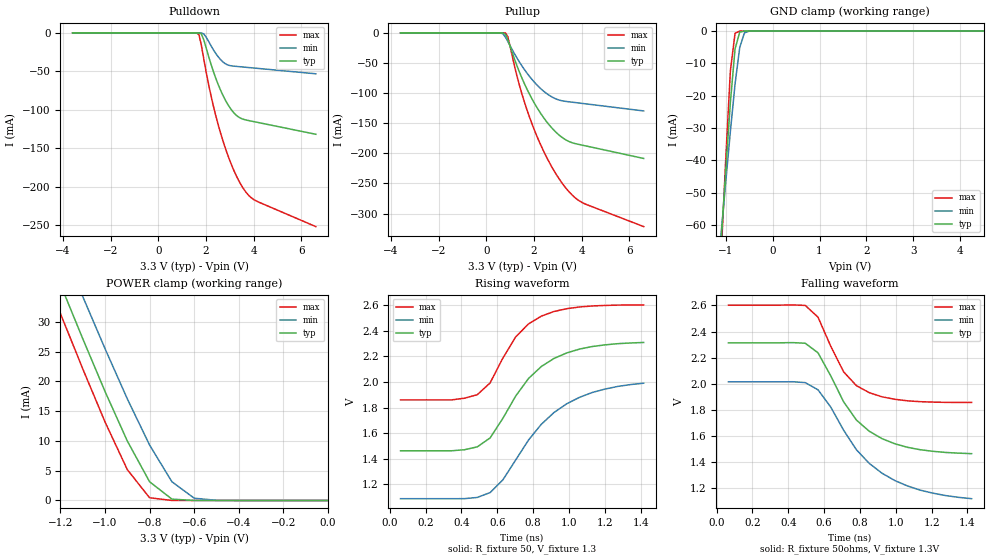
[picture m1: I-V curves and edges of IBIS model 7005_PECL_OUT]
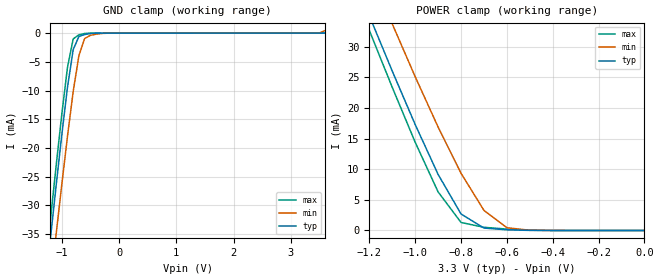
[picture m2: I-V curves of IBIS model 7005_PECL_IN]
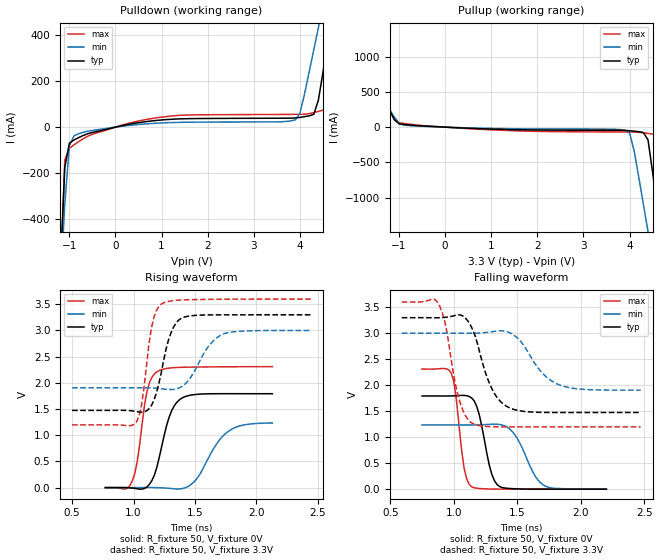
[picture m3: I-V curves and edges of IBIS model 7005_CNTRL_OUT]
|   This file is an IBIS representation of the   |
|   Texas Instruments   |
|   CDC7005   |
|   64 CABGA Package   |
[IBIS Ver]   3.2
[File name]   cdc7005x_02.ibs
[File Rev]   0.2
[Date]   18th of Feb 2004
[Source]   file originated at Texas Instruments
[Notes]   The following information corresponds to the
|   CDC7101 input/output buffers and input ESD structures.
|Revision log: 0.1, 10/02/2002 file released by TEXAS INSTRUMENTS.
|   1- initial version
|   0.2, 02/18/2004 replaced GND Clamp (referenced to VDD), with
|   same plot referenced to GND (0V).
|   Warnings for VT/IV voltage difference relate to truncated
|   VT plots to allow faster simulation frequency if
|   VT time delay is enabled, which is strongly recommended for
|   correct results of the differential PECL buffers. If this is not
|   required, some simulators require to completely disable use of
|   the VT table for better results. If you note problems with
|   differential cross point, it might point to this situation !
[Disclaimer]
(C) Copyright Texas Instruments Incorporated 2001
   All rights reserved
  Texas Instruments Incorporated hereby grants the user of this IBIS
model a non-exclusive, nontransferable license to use this IBIS model
under the following terms.  Before using this IBIS model, the user
should read this license.  If the user does not accept these terms,
the IBIS model should be returned to Texas Instruments within 30 days.
  The user is granted this license only to use the IBIS model and
is not granted rights to sell, load, rent, lease or license the IBIS
model in whole or in part, or in modified form to anyone other than
user.  User may modify the IBIS model to suit its specific applications
but rights to derivative works and such modifications shall belong to
Texas Instruments.
  This IBIS model is provided on an "AS IS" basis and Texas Instruments
makes absolutely no warranty with respect to the information contained
herein.  TEXAS INSTRUMENTS DISCLAIMS AND CUSTOMER WAIVES ALL WARRANTIES,
EXPRESS OR IMPLIED, INCLUDING WARRANTIES OF MERCHANTABILITY OR FITNESS
FOR A PARTICULAR PURPOSE. The entire risk as to quality and performance
is with the Customer. ACCORDINGLY, IN NO EVENT SHALL THE COMPANY BE LIABLE
FOR ANY DAMAGES, WHETHER IN CONTRACT OR TORT,INCLUDING ANY LOST PROFITS
OR OTHER INCIDENTAL, CONSEQUENTIAL, EXEMPLARY, OR PUNITIVE DAMAGES ARISING
OUT OF THE USE OR APPLICATION OF THE IBIS model provided in this package.
Further, Texas Instruments reserves the right to discontinue or make changes
without notice to any product herein to improve reliability, function, or
design. Texas Instruments does not convey any license under patent rights
or any other intellectual property rights, including those of third parties.
Contact Texas Instruments at ATTN: HPA Department,
12500 TI blvd, M/S 8730, Dallas, TX 75243
IBIS Open Forum disclaims all warranties. See DISCLAIM.TXT
in vhdl.org:/pub/IBIS/models for the full disclaimer.
[Copyright]   Copyright 2002, Texas Instruments, All Rights Reserved
[Component]   CDC7005ZVA
[Manufacturer]  Texas Instruments Incorporated
[Package]
| Package paracitics for signal pins only
|   TYP   MIN   MAX
R_pkg   0.197ohms   0.117ohms   0.222ohms
L_pkg   1.790nH   1.335nH   2.000nH
C_pkg   0.600pF   0.506pF   0.675pF
[Pin]   signal_name   model_name   R_Pin   L_Pin   C_Pin
A1   CTRL_LE   7005_SPI_IN   0.200ohms   1.746nH   0.606pF
A2   CTRL_CLK   7005_SPI_IN   0.222ohms   2.000nH   0.597pF
A3   CTRL_DATA   7005_SPI_IN   0.204ohms   1.836nH   0.636pF
A4   CP_OUT   7005_CP_OUT   0.117ohms   1.335nH   0.606pF
A5   OPA_IN   7005_OPA_IN   0.198ohms   1.820nH   0.566pF
A6   OPA_IP   7005_OPA_IN   0.204ohms   1.875nH   0.560pF
A7   OPA_OUT   7005_OPA_OUT   0.134ohms   1.467nH   0.570pF
A8   STATUS_LOCK   7005_CNTRL_OUT   0.199ohms   1.704nH   0.609pF
B1   REF_IN   7005_REF_IN   0.221ohms   1.944nH   0.506pF
|C1   I_REF   7005_IREF   0.203ohms   1.866nH   0.614pF
C8   STATUS_REF   7005_CNTRL_OUT   0.205ohms   1.826nH   0.556pF
D1   VCXO_IN   7005_PECL_IN   0.197ohms   1.803nH   0.675pF
D8   STATUS_VCOX   7005_CNTRL_OUT   0.195ohms   1.763nH   0.557pF
E1   VCXO_IN_B   7005_PECL_IN   0.200ohms   1.826nH   0.658pF
F1   Y0   7005_PECL_OUT   0.206ohms   1.854nH   0.600pF
F8   Y4B   7005_PECL_OUT   0.202ohms   1.849nH   0.601pF
G1   Y0B   7005_PECL_OUT   0.211ohms   1.886nH   0.607pF
G8   Y4   7005_PECL_OUT   0.208ohms   1.767nH   0.522pF
H1   NPD   7005_LOGIC_IN   0.199ohms   1.736nH   0.604pF
H2   Y1   7005_PECL_OUT   0.205ohms   1.874nH   0.638pF
H3   Y1B   7005_PECL_OUT   0.189ohms   1.736nH   0.606pF
H4   Y2   7005_PECL_OUT   0.200ohms   1.835nH   0.623pF
H5   Y2B   7005_PECL_OUT   0.201ohms   1.843nH   0.607pF
H6   Y3   7005_PECL_OUT   0.204ohms   1.882nH   0.619pF
H7   Y3B   7005_PECL_OUT   0.208ohms   1.898nH   0.647pF
H8   NRESET   7005_LOGIC_IN   0.203ohms   1.571nH   0.601pF
| equivilant summary for balls: C3,C4,C5,C6,C7 and C7
C3   AVCC_all   Power   0.034ohms   0.319nH   2.076pF
| equivilant summary for balls: B2,B3,B4,B5,B6,B7,B8,C2,D2,D3,D4,D5,D6
|   E2,F2,F3,F4,F5,F6
B2   GND_all   GND   0.008ohms   0.069nH   7.236pF
| equivilant summary for balls: D7,E3,E4,E5,E6,E7,E8,F7,G2,G3,G4,G5,G6,G7
D7   VCC_all   Power   0.011ohms   0.099nH   4.810pF
[Diff_Pin]  inv_pin  vdiff   tdelay_typ  tdelay_min  tdelay_max
F1   G1   0V   0ns   0ns   0ns   | Y0+ / Y0-
H2   H3   0V   0ns   0ns   0ns   | Y1+ / Y1-
H4   H5   0V   0ns   0ns   0ns   | Y2+ / Y2-
H6   H7   0V   0ns   0ns   0ns   | Y3+ / Y3-
G8   F8   0V   0ns   0ns   0ns   | Y4+ / Y4-
D1   E1   0.5V   0ns   0ns   0ns   | VCXO_IN+ / VCXO_IN-
A6   A5   0.1V   0ns   0ns   0ns   | OPA_IP / OPA_IN
[Model Selector]   7005_CP_OUT
7005_CP_DOWN   negative_pulse_2mA
7005_CP_UP   positive_pulse_2mA
| Models and submodels in the file (10): 7005_PECL_OUT (3-state_ECL), 7005_PECL_IN (Input), 7005_CNTRL_OUT (Output), 7005_REF_IN (Input), 7005_SPI_IN (Input), 7005_LOGIC_IN (Input), 7005_OPA_OUT (Output), 7005_OPA_IN (Input), 7005_CP_UP (3-state), 7005_CP_DOWN (3-state)
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|   Differential Output Driver MODEL
[Model]   7005_PECL_OUT
Model_type   3-state_ECL
| Signals   Y0, Y0B, Y1, Y1B, Y2, Y2B, Y3, Y3B, Y4, Y4B
Vmeas = 1.89V   |Vref for timing measurments
Cref = 0pF   |c_load for timing spec
Rref = 50   |R_load for timing spec
Vref = 1.3V   |Timing spec test load voltage
| variable   typ   min   max
C_comp   1.6pF   1.2pF   2.2pF
[Temperature Range]   27   125   -20
[Voltage range]   3.3V   3.0V   3.6V
[Pulldown reference]   3.3V   3.0V   3.6V
[GND Clamp reference]   0V   0V   0V
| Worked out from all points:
|   GND clamp passes 1 mA (typ) near -0.71 V on its own axis
|   POWER clamp passes 1 mA (typ) near -0.73 V on its own axis
|   rising waveform, R_fixture 50, V_fixture 1.3: 20-80 % time 275ps typ, 321ps min, 209ps max; typ from 1.46 V to 2.31 V
|   falling waveform, R_fixture 50ohms, V_fixture 1.3V: 20-80 % time 251ps typ, 314ps min, 183ps max; typ from 2.31 V to 1.47 V
[Pullup]
|   27C:3.3V:nominal   125C:3.0V:weak   -20C:3.6V:strong
|  Voltage   I(typ)   I(min)   I(max)
-3.6V     437pA      8.06nA     324.7pA
500mV     -84.04nA   -11.65uA   -371.3pA
700mV     -101.2uA   -1.872mA   -2.864uA
800mV     -2.246mA   -7.123mA   -226.3uA
900mV     -11.06mA   -14.21mA   -6.425mA
1.4V      -66.31mA   -49.24mA   -88.69mA
1.9V      -108.6mA   -76.68mA   -149.5mA
2.5V      -146mA     -99.87mA   -204.2mA
3.2V      -174.2mA   -112.9mA   -250.6mA
3.6V      -182.4mA   -115.1mA   -269.2mA
4V        -186.2mA   -117mA     -281.2mA
6.6V      -208.5mA   -129.6mA   -321.5mA
[Pulldown]
|   27C:3.3V:nominal   125C:3.0V:weak   -20C:3.6V:strong
|   Voltage   I(typ)   I(min)   I(max)
-3.6V     280.9pA    304.5pA    264.7pA
1.6V      -1.679uA   -521.3nA   -43.83uA
1.7V      -58.05uA   -8.476uA   -2.396mA
1.8V      -1.47mA    -132uA     -16mA
1.9V      -8.843mA   -1.407mA   -33.6mA
2.2V      -40.32mA   -16.53mA   -81.03mA
2.5V      -66.73mA   -30.89mA   -118.8mA
3V        -97.48mA   -42.66mA   -166.6mA
3.5V      -111.8mA   -44.34mA   -199.5mA
3.8V      -114.3mA   -45.21mA   -211.9mA
4.1V      -116.2mA   -46.08mA   -218.7mA
6.6V      -132mA     -53.32mA   -252.1mA
[GND Clamp]
|   27C:3.3V:nominal   125C:3.0V:weak   -20C:3.6V:strong
|   Voltage   I(typ)   I(min)   I(max)
-3.6V     -846.1mA   -726mA     -1.01A
-1.1V     -65.74mA   -63.12mA   -70.56mA
-1V       -43.58mA   -46.98mA   -40.08mA
-900mV    -22.15mA   -31.16mA   -12.38mA
-800mV    -5.529mA   -16.41mA   -692.9uA
-700mV    -333.5uA   -5.056mA   -8.688uA
-600mV    -9.161uA   -575uA     -94.39nA
-500mV    -237.2nA   -35.55uA   -1.21nA
6.6V      452.4pA    471.7pA    424.6pA
[POWER Clamp]
|   27C:3.3V:nominal   125C:3.0V:weak   -20C:3.6V:strong
|  Voltage   I(typ)   I(min)   I(max)
-3.6V     263.5mA    264.3mA    263.5mA
-1.3V     45.57mA    52.26mA    40.83mA
-1.2V     36.3mA     43.2mA     31.38mA
-1.1V     27.17mA    34.25mA    22.11mA
-1V       18.31mA    25.49mA    13.19mA
-900mV    9.992mA    17.07mA    5.178mA
-800mV    3.144mA    9.308mA    454.2uA
-700mV    228.8uA    3.147mA    5.697uA
-600mV    6.116uA    387.4uA    58.55nA
-500mV    150.9nA    23.42uA    752.7pA
0V        84.38pA    102.7pA    89.81pA
[ramp]
| variable   typ   min   max
dV/dt_r   0.5117/2.7842E-10   0.5571/3.3895E-10   0.4456/2.0819E-10
dV/dt_f   0.5117/2.5529E-10   0.5571/3.4568E-10   0.4456/1.8152E-10
[Rising Waveform]
R_fixture = 50
V_fixture =  1.3
V_fixture_min = 1.0
V_fixture_max = 1.6  | Plot was truncated to
|   allow shorter simulation periodes.
|   27C:3.3V:nominal   125C:3.0V:weak  -20C:3.6V:strong
|   Time   V(typ)   V(min)   V(max)
59.71ps   1.462V     1.087V     1.86V
416.9ps   1.47V      1.087V     1.873V
488.3ps   1.492V     1.096V     1.901V
559.7ps   1.562V     1.134V     1.993V
631.1ps   1.716V     1.234V     2.188V
702.6ps   1.89V      1.39V      2.353V
845.4ps   2.121V     1.669V     2.515V
916.9ps   2.185V     1.762V     2.552V
1.06ns    2.258V     1.881V     2.588V
1.417ns   2.31V      1.991V     2.603V
[Falling Waveform]
R_fixture = 50ohms
V_fixture =  1.3V
V_fixture_min = 1.0V
V_fixture_max = 1.6V   |  Plot was truncated to
|   allow shorter simulation periodes.
|   27C:3.3V:nominal   125C:3.0V:weak -20C:3.6V:strong
|   Time   V(typ)   V(min)   V(max)
65.71ps   2.314V     2.015V     2.602V
494.3ps   2.311V     2.01V      2.6V
565.7ps   2.238V     1.955V     2.51V
637.1ps   2.061V     1.822V     2.287V
708.6ps   1.863V     1.645V     2.092V
780ps     1.723V     1.496V     1.987V
922.9ps   1.581V     1.316V     1.901V
1.066ns   1.514V     1.218V     1.87V
1.209ns   1.484V     1.163V     1.86V
1.423ns   1.466V     1.121V     1.858V
|   Differential Input Receiver Model
[Model]   7005_PECL_IN
Model_type   Input
Polarity   Non-Inverting
Enable   Active-High
Vinl = 1.6575V   | PECL levels refer to VDD. 3.3-(1.81+1.475)/2
Vinh = 2.2775V   |   3.3-(1.165+.088)/2
|   typ   min   max
C_comp   0.21pF   NA   NA
[Temperature range]   27   125   -20
[Voltage range]   3.3   3.0   3.6
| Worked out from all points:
|   GND clamp passes 1 mA (typ) near -0.72 V on its own axis
|   POWER clamp passes 1 mA (typ) near -0.73 V on its own axis
| Notes: (1) Vtable = Vcc - Voutput
|   (2) Pullup data includes the effects of the clamping circuitry
[POWER Clamp]
|   27C:3.3V:nominal   125C:3.0V:weak   -20C:3.6V:strong
|  Voltage   I(typ)   I(min)   I(max)
-3.6V     265.8mA    263.4mA    273.1mA
-1.2V     35.02mA    42.56mA    32.64mA
-1.1V     26mA       33.7mA     23.35mA
-1V       17.28mA    25.09mA    14.39mA
-900mV    9.15mA     16.88mA    6.291mA
-800mV    2.691mA    9.338mA    1.306mA
-700mV    397uA      3.282mA    517.8uA
-600mV    106.3uA    454.8uA    227uA
-500mV    15.87uA    36.77uA    48.73uA
0V        85.66pA    160pA      90.57pA
[GND Clamp]
|   27C:3.3V:nominal   125C:3.0V:weak   -20C:3.6V:strong
|  Voltage   I(typ)   I(min)   I(max)
-3.6V     -268.1mA   -268.4mA   -271.2mA
-1.3V     -45.38mA   -53.26mA   -42.38mA
-1.2V     -35.99mA   -44.19mA   -32.76mA
-1.1V     -26.76mA   -35.23mA   -23.31mA
-1V       -17.81mA   -26.44mA   -14.21mA
-900mV    -9.461mA   -17.98mA   -5.998mA
-800mV    -2.874mA   -10.17mA   -1.017mA
-700mV    -575.1uA   -3.894mA   -292.2uA
-600mV    -252.8uA   -947.5uA   -69.37uA
-300mV    -10.26uA   -59.25uA   -7.753uA
3.4V      131.5pA    2.975uA    79.13pA
3.6V      47.15nA    454.8uA    90.57pA
|   Device Control Output Driver Model
[Model]   7005_CNTRL_OUT
Model_type   Output
Polarity   Non-Inverting
Enable   Active-High
Vmeas = 0.9V   |Vref for timing measurements.
Cref = 0pF   |load capacitance for timing spec.
Rref = 50ohms   |50 Ohm to GND (VCC)
Vref = 0V   |Timing specification test load voltage; GND
|   typ   min   max
C_comp   1.84pF   NA   NA
[Temperature range]   27   125   -20
[Voltage range]   3.3   3.0   3.6
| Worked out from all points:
|   slope of the pulldown table from 0 to 0.495 V, typ, clamps not added: 25.5 ohm
|   slope of the pullup table from 0 to 0.495 V, typ, clamps not added: 32.4 ohm
|   rising waveform, R_fixture 50, V_fixture 0V: 20-80 % time 119ps typ, 192ps min, 83.9ps max; typ from 0 V to 1.79 V
|   falling waveform, R_fixture 50, V_fixture 0V: 20-80 % time 90.9ps typ, 146ps min, 64.9ps max; typ from 1.79 V to 0 V
|   rising waveform, R_fixture 50, V_fixture 3.3V: 20-80 % time 112ps typ, 171ps min, 81.9ps max; typ from 1.47 V to 3.3 V
|   falling waveform, R_fixture 50, V_fixture 3.3V: 20-80 % time 150ps typ, 200ps min, 110ps max; typ from 3.3 V to 1.48 V
| Notes: (1) Vtable = Vcc - Voutput
|   (2) Pullup data includes the effects of the ESD
|   clamping circuitry
[Pullup]
|   27C:3.3V:nominal   125C:3.0V:weak   -20C:3.6V:strong
|  Voltage   I(typ)   I(min)   I(max)
-3.6V     3.231A     2.546A     4.154A
-2.5V     1.856A     1.489A     2.366A
-2.2V     1.481A     1.2A       1.879A
-1.9V     1.106A     911.7mA    1.391A
-1V       46.45mA    58.48mA    62.25mA
3.9V      -46.72mA   -42.31mA   -68.83mA
4.1V      -57.23mA   -338.9mA   -70mA
4.4V      -181.6mA   -1.482A    -89.55mA
4.6V      -1.142A    -2.251A    -112mA
4.7V      -1.642A    -2.636A    -160.1mA
4.9V      -2.642A    -3.405A    -1.365A
6.6V      -11.14A    -9.943A    -12.41A
[Pulldown]
|   27C:3.3V:nominal   125C:3.0V:weak   -20C:3.6V:strong
|  Voltage   I(typ)   I(min)   I(max)
-3.6V     -12.64A    -9.941A    -16.3A
-1.2V     -638mA     -710.4mA   -698.9mA
-1.1V     -176.9mA   -336.1mA   -142.9mA
-1V       -69.89mA   -80.95mA   -92.23mA
-900mV    -56.15mA   -37.94mA   -77.1mA
900mV     29.4mA     17.24mA    40.92mA
3.9V      40.02mA    31.45mA    55.55mA
4V        42.48mA    60.4mA     55.69mA
4.4V      117.5mA    432.9mA    68.4mA
4.7V      489.8mA    721.3mA    115.4mA
4.9V      739.8mA    913.6mA    433.4mA
6.6V      2.865A     2.548A     3.196A
[ramp]
| variable   typ   min   max
dV/dt_r   1.0759/1.1902E-10   0.7405/1.9176E-10   1.3856/8.3905E-11
dV/dt_f   1.0759/9.0932E-11   0.7405/1.4575E-10   1.3856/6.4836E-11
[Rising Waveform]
R_fixture = 50
V_fixture = 0V
|   27C:3.3V:nominal   125C:3.0V:weak  -20C:3.6V:strong
|   Time   V(typ)   V(min)   V(max)
770.2ps   -100uV     0V         1mV
990.2ps   -9mV       300uV      127.7mV
1.03ns    -20.3mV    800uV      498mV
1.11ns    14.6mV     2mV        1.841V
1.19ns    391.7mV    -400uV     2.211V
1.29ns    1.346V     -13mV      2.282V
1.39ns    1.704V     -21.2mV    2.297V
1.51ns    1.779V     157.1mV    2.302V
1.77ns    1.793V     1.072V     2.307V
2.13ns    1.793V     1.234V     2.309V
[Falling Waveform]
R_fixture = 50
V_fixture = 0V
|   27C:3.3V:nominal   125C:3.0V:weak  -20C:3.6V:strong
|   Time   V(typ)   V(min)   V(max)
750ps     1.793V     1.236V     2.31V
980ps     1.794V     1.236V     2.235V
1.02ns    1.798V     1.235V     1.724V
1.08ns    1.804V     1.235V     419.2mV
1.14ns    1.756V     1.235V     46.3mV
1.2ns     1.433V     1.238V     13.9mV
1.3ns     277.9mV    1.25V      2.6mV
1.36ns    50.6mV     1.244V     1.1mV
1.7ns     600uV      87.7mV     300uV
2.2ns     200uV      500uV      300uV
[Rising Waveform]
R_fixture = 50
V_fixture =  3.3V
V_fixture_min = 3.0
V_fixture_max = 3.6
|   27C:3.3V:nominal   125C:3.0V:weak  -20C:3.6V:strong
|   Time   V(typ)   V(min)   V(max)
500ps     1.474V     1.905V     1.198V
1.025ns   1.452V     1.906V     1.258V
1.065ns   1.441V     1.906V     1.575V
1.145ns   1.565V     1.903V     3.036V
1.185ns   1.8V       1.897V     3.373V
1.245ns   2.425V     1.882V     3.528V
1.325ns   3.061V     1.875V     3.571V
1.405ns   3.25V      1.949V     3.584V
1.725ns   3.299V     2.927V     3.596V
2.445ns   3.299V     3.001V     3.6V
[Falling Waveform]
R_fixture = 50
V_fixture =  3.3V
V_fixture_min = 3.0
V_fixture_max = 3.6
|   27C:3.3V:nominal   125C:3.0V:weak  -20C:3.6V:strong
|   Time   V(typ)   V(min)   V(max)
590.3ps   3.299V     3.001V     3.601V
870.3ps   3.297V     3.001V     3.602V
930.3ps   3.304V     3.001V     3.214V
1.01ns    3.342V     3V         2.051V
1.05ns    3.352V     2.999V     1.659V
1.15ns    3.061V     2.999V     1.262V
1.29ns    1.981V     3.024V     1.204V
1.43ns    1.575V     3.02V      1.198V
1.81ns    1.475V     2.027V     1.198V
2.47ns    1.475V     1.905V     1.198V
